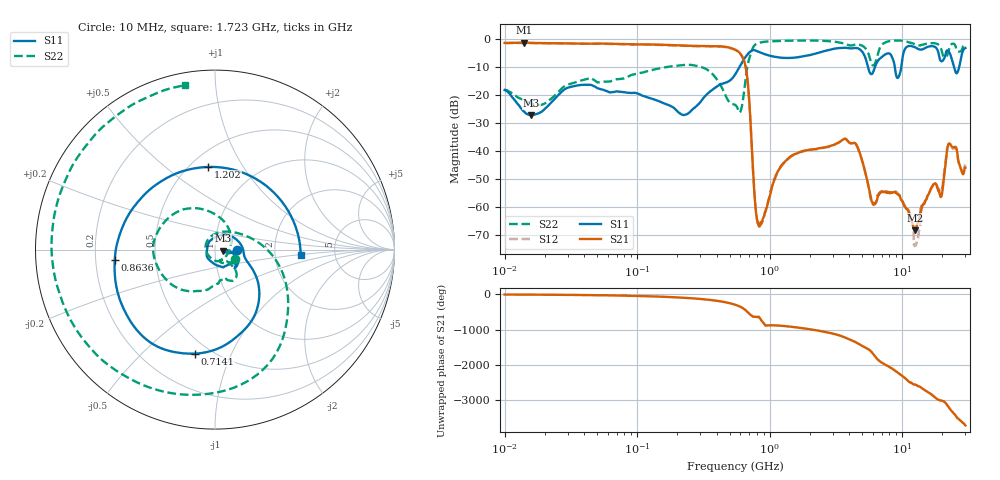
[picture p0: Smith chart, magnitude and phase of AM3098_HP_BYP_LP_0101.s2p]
!Agilent Technologies,E8364B,MY43040894,A.07.50.67
!Agilent E8364B: A.07.50.67
!Date: Wednesday, June 17, 2020 09:20:08
!Correction: S11(Full 2 Port(1,2))
!S21(Full 2 Port(1,2))
!S12(Full 2 Port(1,2))
!S22(Full 2 Port(1,2))
!S2P File: Measurements: S11, S21, S12, S22:Log Frequency Sweep
# Hz S  dB  R 50
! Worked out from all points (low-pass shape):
!   1601 points, 10 MHz to 30 GHz, reference 50 ohm
!   highest |S21| = -1.40 dB at 14.05 MHz (marker M1); lowest = -68.2 dB at 12.5 GHz (marker M2)
!   |S21| within 3 dB of the highest: start of sweep to 574.8 MHz
!   lowest |S11| = -27.2 dB at 15.93 MHz (marker M3), VSWR 1.09, Z = 54.5 - j0.653 ohm
!   |S11| at or under -10 dB: 5.512 GHz to 6.239 GHz (727.9 MHz wide, 12.4 % of centre); 8.799 GHz to 9.855 GHz (1.056 GHz wide, 11.3 % of centre); 24.6 GHz to 26.94 GHz (2.337 GHz wide, 9.07 % of centre)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
!   |S22| runs from -26.3 to -0.6 dB; largest |S21 - S12| = 0.02
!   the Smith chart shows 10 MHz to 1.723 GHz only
!   S11 on the Smith chart (normalised r, x): 10 MHz: 1.28, -0.01; 714.1 MHz: 0.41, -0.74; 863.6 MHz: 0.28, -0.05; 1.202 GHz: 0.61, +0.71; 1.723 GHz: 2.82, -0.22
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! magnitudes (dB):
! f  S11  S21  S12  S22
! 10 MHz  -18.2  -1.4  -1.6  -18.2
! 14.05 MHz  -26.0  -1.4  -1.5  -21.9
! 15.93 MHz  -27.2  -1.5  -1.5  -23.1
! 38.04 MHz  -16.4  -1.7  -1.7  -14.8
! 144.7 MHz  -22.2  -2.1  -2.1  -10.6
! 232.8 MHz  -27.1  -2.4  -2.5  -9.3
! 547.7 MHz  -12.8  -3.9  -3.9  -23.5
! 652.6 MHz  -6.7  -9.1  -9.1  -15.7
! 714.1 MHz  -4.6  -28.0  -28.0  -5.9
! 789.2 MHz  -4.3  -61.9  -61.9  -1.9
! 863.6 MHz  -5.0  -65.7  -66.0  -1.3
! 1.202 GHz  -6.7  -45.7  -46.0  -0.7
! 1.723 GHz  -6.4  -40.2  -40.3  -0.6
! 2.084 GHz  -5.6  -39.5  -39.4  -0.6
! 4.391 GHz  -3.3  -37.1  -37.3  -2.1
! 5.989 GHz  -12.2  -58.3  -58.8  -9.4
! 7.926 GHz  -5.2  -54.8  -54.6  -0.9
! 9.302 GHz  -13.9  -55.5  -55.2  -0.7
! 12.5 GHz  -3.0  -68.2  -73.7  -2.0
! 19.7 GHz  -8.0  -56.2  -54.4  -3.7
! 22.56 GHz  -4.6  -37.3  -37.7  -3.7
! 30 GHz  -3.3  -45.9  -44.8  -2.4
